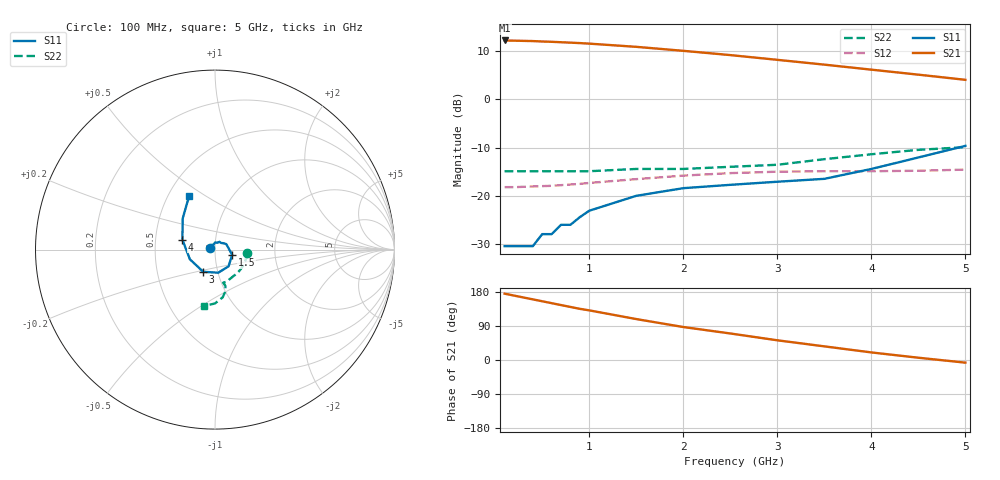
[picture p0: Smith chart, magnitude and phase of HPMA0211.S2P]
! HPMA-0211
! Typical S-Parameters, Z  = 50 , T  = 25 C, I  = 25mA
# ghz s ma r 50
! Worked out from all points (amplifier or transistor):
!   18 points, 100 MHz to 5 GHz, reference 50 ohm
!   highest |S21| = 12.3 dB at 100 MHz (marker M1)
!   |S21| within 3 dB of that: start of sweep to 2.479 GHz
!   unconditionally stable (mu >= 1): start of sweep to end of sweep
!   at 400 MHz: K = 1.21, MAG = 12.3 dB, |S12| = -18.1 dB
!   at 1 GHz: K = 1.20, MAG = 11.7 dB, |S12| = -17.3 dB
!   at 5 GHz: K = 1.38, MAG = 5.6 dB, |S12| = -14.6 dB
!   S11 on the Smith chart (normalised r, x): 100 MHz: 0.94, +0.02; 1.5 GHz: 1.21, -0.07; 3 GHz: 0.85, -0.21; 4 GHz: 0.69, +0.08; 5 GHz: 0.64, +0.42
0.1  0.03 160.0  4.1 175.0  0.123 1.0  0.18 -6.0
0.2  0.03 141.0  4.08 170.0  0.123 3.0  0.18 -13.0
0.3  0.03 121.0  4.06 165.0  0.124 4.0  0.18 -20.0
0.4  0.03 104.0  4.04 160.0  0.125 5.0  0.18 -26.0
0.5  0.04 88.0  4 155.0  0.126 6.0  0.18 -31.0
0.6  0.04 73.0  3.97 150.0  0.127 7.0  0.18 -37.0
0.7  0.05 60.0  3.93 145.0  0.129 8.0  0.18 -42.0
0.8  0.05 48.0  3.89 140.0  0.131 9.0  0.18 -47.0
0.9  0.06 36.0  3.85 135.0  0.133 10.0  0.18 -52.0
1  0.07 26.0  3.8 131.0  0.136 10.0  0.18 -56.0
1.5  0.1 -17.0  3.52 108.0  0.149 13.0  0.19 -70.0
2  0.12 -51.0  3.2 87.0  0.162 12.0  0.19 -76.0
2.5  0.13 -82.0  2.89 70.0  0.172 12.0  0.2 -75.0
3  0.14 -118.0  2.58 52.0  0.178 9.0  0.21 -74.0
3.5  0.15 -159.0  2.3 36.0  0.18 7.0  0.24 -76.0
4  0.19 163.0  2.04 20.0  0.18 6.0  0.27 -81.0
4.5  0.25 136.0  1.81 6.0  0.182 7.0  0.3 -90.0
5  0.33 116.0  1.6 -7.0  0.187 8.0  0.32 -101.0
